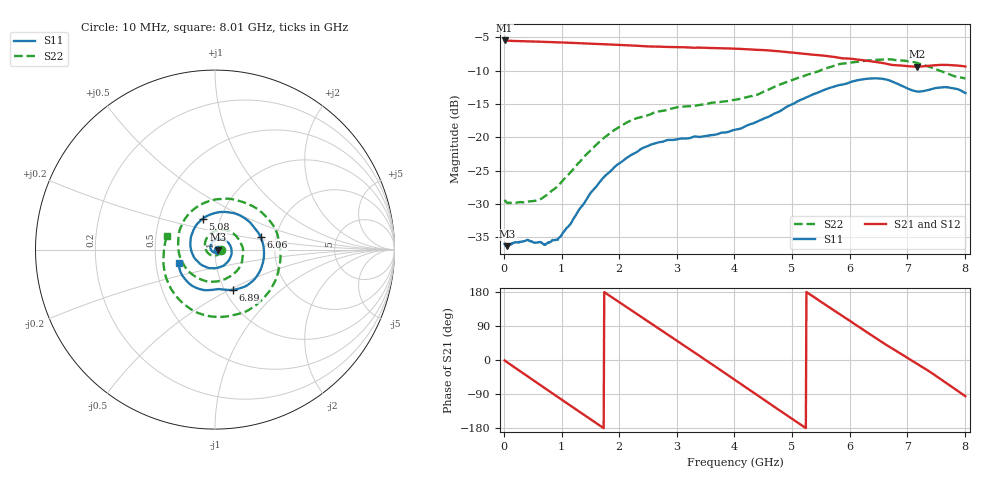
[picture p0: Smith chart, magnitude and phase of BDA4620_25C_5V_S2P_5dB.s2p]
!Agilent Technologies,E5071B,MY42404982,A.09.10
!Date: Wed May 06 08:59:09 2026
!Data & Calibration Information:
!Freq	S11:SOLT2(ON)	S21:SOLT2(ON)	S12:SOLT2(ON)	S22:SOLT2(ON)
# Hz S RI R 50
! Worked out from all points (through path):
!   801 points, 10 MHz to 8.01 GHz, reference 50 ohm
!   highest |S21| = -5.45 dB at 10 MHz (marker M1); lowest = -9.4 dB at 7.17 GHz (marker M2)
!   group delay of S21, straight-line fit = 283 ps
!   lowest |S11| = -36.3 dB at 60 MHz (marker M3), VSWR 1.03, Z = 51.5 - j0.131 ohm
!   |S11| at or under -10 dB: start of sweep to end of sweep
!   |S22| runs from -29.8 to -8.3 dB; largest |S21 - S12| = 0.0022
!   S11 on the Smith chart (normalised r, x): 10 MHz: 1.03, -0.00; 5.08 GHz: 0.82, +0.29; 6.06 GHz: 1.66, +0.25; 6.89 GHz: 1.09, -0.52; 8.01 GHz: 0.66, -0.10
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1e7  0.0159 -0.000975  0.5337 -0.0114  0.5347 -0.0117  0.0339 -0.00266
6e7  0.0152 -0.00127  0.5282 -0.0608  0.5294 -0.0617  0.0319 -0.00566
3.7e8  0.0138 -0.00954  0.4089 -0.3312  0.4092 -0.3321  0.0188 -0.0267
7.3e8  0.000149 -0.0159  0.1213 -0.5063  0.121 -0.5068  -0.0164 -0.0329
1.03e9  -0.0175 -0.00833  -0.1561 -0.4906  -0.1567 -0.4911  -0.0473 -0.00888
1.35e9  -0.0261 0.0158  -0.394 -0.3214  -0.3941 -0.3221  -0.0548 0.0406
1.64e9  -0.0146 0.0425  -0.4951 -0.0821  -0.4958 -0.0822  -0.0269 0.0872
1.94e9  0.0159 0.059  -0.4613 0.1802  -0.4622 0.1804  0.0333 0.1106
2.33e9  0.0644 0.0457  -0.2339 0.4264  -0.2342 0.4272  0.119 0.0743
2.68e9  0.0919 0.00124  0.0551 0.4765  0.0556 0.4769  0.1564 -0.00696
3e9  0.0826 -0.0502  0.3002 0.37  0.3005 0.3699  0.1388 -0.0948
3.39e9  0.0351 -0.0947  0.4622 0.0917  0.4627 0.0913  0.0442 -0.169
4.01e9  -0.0787 -0.0826  0.2811 -0.368  0.2805 -0.3686  -0.1604 -0.105
4.51e9  -0.137 0.0189  -0.1126 -0.4377  -0.1135 -0.438  -0.2011 0.0923
5.08e9  -0.0693 0.171  -0.4116 -0.1233  -0.4125 -0.1226  -0.00721 0.2778
5.35e9  0.0202 0.2081  -0.4106 0.078  -0.4104 0.0786  0.1328 0.2716
6.06e9  0.2538 0.0714  -0.051 0.3841  -0.0504 0.3848  0.3657 -0.0242
6.68e9  0.1834 -0.1966  0.2869 0.206  0.2885 0.2057  0.1882 -0.3363
6.89e9  0.1013 -0.2245  0.3324 0.0964  0.3333 0.0956  0.0632 -0.3725
7.17e9  0.0224 -0.22  0.3342 -0.0576  0.3351 -0.0589  -0.1135 -0.3441
7.57e9  -0.0973 -0.2158  0.228 -0.2658  0.2281 -0.2667  -0.2684 -0.1673
8.01e9  -0.2018 -0.0754  -0.033 -0.3387  -0.0338 -0.3398  -0.2663 0.0762
